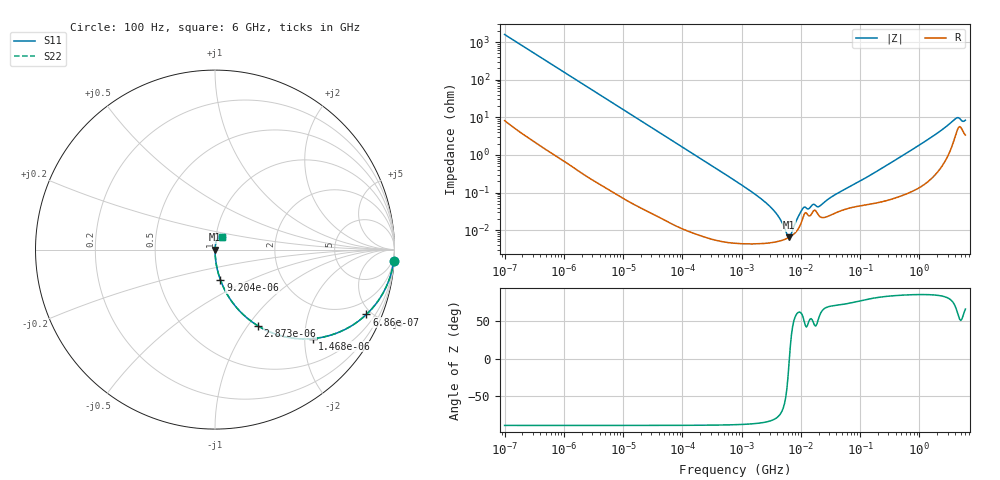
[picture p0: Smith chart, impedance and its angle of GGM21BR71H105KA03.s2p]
!Murata Part Number: GGM21BR71H105KA03
!These Parameters are Measured in Series Mode Connection
!Data Generated on Jun 19, 2026
!  o--ll--o
!Port1  Port2
!  o------o
!Operation Temp=25[degC], DC Bias Voltage=0[V]
!Freq. Start=100[Hz] Stop=6[GHz] 401[Steps]
# Hz S RI R 50
!Freq.(Hz) S11(Real) S11(Imag) S21(Real) S21(Imag) S12(Real) S12(Imag) S22(Real) S22(Imag)
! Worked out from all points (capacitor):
!   401 points, 100 Hz to 6 GHz, reference 50 ohm
!   read as one part in series: C = 999 nF near 109 Hz
!   lowest |Z| = 6.46 mohm at 6.353 MHz (marker M1)
!   series resonance near 6.412 MHz, so ESL is about 620 pH
!   S11 on the Smith chart (normalised r, x): 100 Hz: 1, -32; 686 Hz: 1.02, -4.66; 1.468 kHz: 1.01, -2.18; 2.873 kHz: 1.00, -1.12; 9.204 kHz: 1.00, -0.35; 6 GHz: 1.07, +0.15
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100  0.9957 -0.0626  0.00425 0.0626  0.00425 0.0626  0.9957 -0.0626
335  0.957 -0.2007  0.043 0.2007  0.043 0.2007  0.957 -0.2007
686  0.8436 -0.3611  0.1564 0.3611  0.1564 0.3611  0.8436 -0.3611
1468  0.5435 -0.496  0.4565 0.496  0.4565 0.496  0.5435 -0.496
2008  0.3898 -0.4857  0.6102 0.4857  0.6102 0.4857  0.3898 -0.4857
2873  0.2387 -0.4243  0.7613 0.4243  0.7613 0.4243  0.2387 -0.4243
9204  0.0304 -0.1695  0.9696 0.1695  0.9696 0.1695  0.0304 -0.1695
40335  0.00182 -0.04  0.9982 0.04  0.9982 0.04  0.00182 -0.04
774597  4.9e-05 -0.00207  1 0.00207  1 0.00207  4.9e-05 -0.00207
2837864  4.56e-05 -0.000465  1 0.000465  1 0.000465  4.56e-05 -0.000465
4060267  4.98e-05 -0.000244  1 0.000244  1 0.000244  4.98e-05 -0.000244
5554849  5.81e-05 -7.55e-05  0.9999 7.55e-05  0.9999 7.55e-05  5.81e-05 -7.55e-05
6353432  6.44e-05 -4.8e-06  0.9999 4.8e-06  0.9999 4.8e-06  6.44e-05 -4.8e-06
7266822  7.39e-05 6.81e-05  0.9999 -6.81e-05  0.9999 -6.81e-05  7.39e-05 6.81e-05
1.087309e7  0.000214 0.000317  0.9998 -0.000317  0.9998 -0.000317  0.000214 0.000317
1.555665e7  0.000287 0.000367  0.9997 -0.000367  0.9997 -0.000367  0.000287 0.000367
2.128304e7  0.000226 0.000386  0.9998 -0.000386  0.9998 -0.000386  0.000226 0.000386
3.64232e7  0.000276 0.000798  0.9997 -0.000798  0.9997 -0.000798  0.000276 0.000798
3.124326e8  0.000673 0.00581  0.9993 -0.00581  0.9993 -0.00581  0.000673 0.00581
1.637704e9  0.00332 0.0301  0.9967 -0.0301  0.9967 -0.0301  0.00332 0.0301
4.009986e9  0.0356 0.0797  0.9644 -0.0797  0.9644 -0.0797  0.0356 0.0797
6e9  0.0379 0.0714  0.9621 -0.0714  0.9621 -0.0714  0.0379 0.0714
